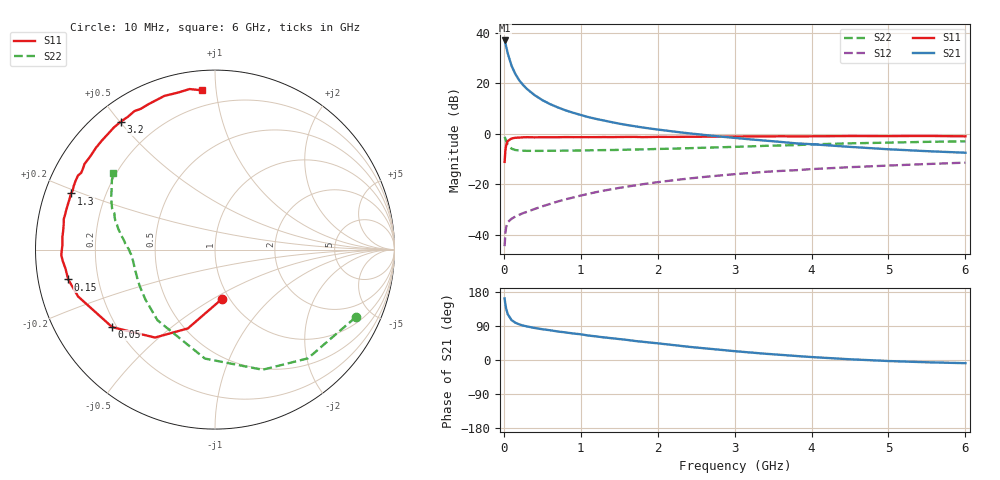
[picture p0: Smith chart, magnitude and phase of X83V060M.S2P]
! SIEMENS Small Signal Semiconductors
! BFP136W
! Si NPN RF Bipolar Junction Transistor in SOT343
! VCE = 3 V  IC = 60 mA
! Common Emitter S-Parameters:  September  1994
# GHz  S  MA  R  50
!  f  S11  S21  S12  S22
! GHz  MAG  ANG  MAG  ANG  MAG  ANG  MAG  ANG
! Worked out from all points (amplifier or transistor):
!   40 points, 10 MHz to 6 GHz, reference 50 ohm
!   highest |S21| = 36.9 dB at 10 MHz (marker M1)
!   |S21| within 3 dB of that: start of sweep to 34.86 MHz
!   unconditionally stable (mu >= 1): 594.7 MHz to 2.885 GHz
!   at 200 MHz: K = 0.59, MSG = 26.6 dB, |S12| = -32.0 dB
!   at 1.5 GHz: K = 1.10, MAG = 10.8 dB, |S12| = -21.4 dB
!   at 6 GHz: K = 0.96, MSG = 2.0 dB, |S12| = -11.4 dB
!   S11 on the Smith chart (normalised r, x): 10 MHz: 0.92, -0.55; 50 MHz: 0.18, -0.32; 150 MHz: 0.09, -0.10; 1.3 GHz: 0.08, +0.19; 3.2 GHz: 0.08, +0.50; 6 GHz: 0.11, +0.92
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0.01  0.278 -82.1  69.91 162.3  0.006 72.6  0.8694 -25.7
0.02  0.4645 -109.0  61.72 147.1  0.0108 60.3  0.7969 -49.5
0.03  0.5932 -124.3  53.35 135.8  0.0143 51.5  0.72 -68.4
0.05  0.7175 -143.0  39.19 121.1  0.0178 40.2  0.6097 -95.3
0.1  0.8063 -161.1  22.14 105.3  0.0209 33.4  0.5075 -129.2
0.15  0.8345 -168.5  15.15 98.3  0.0231 35.1  0.477 -144.5
0.2  0.8395 -172.7  11.41 94.0  0.025 36.7  0.4671 -152.8
0.25  0.851 -175.8  9.205 90.9  0.027 38.7  0.4632 -158.1
0.3  0.857 -178.0  7.703 88.6  0.0286 41.0  0.4599 -161.8
0.4  0.8504 178.1  5.804 84.5  0.0326 45.5  0.4592 -166.6
0.5  0.8532 175.3  4.629 81.2  0.0368 48.8  0.4596 -169.7
0.6  0.8524 173.2  3.864 78.5  0.041 51.5  0.4606 -171.7
0.7  0.8545 170.6  3.326 75.3  0.0458 53.9  0.4622 -173.1
0.9  0.8576 166.8  2.604 70.1  0.0549 56.1  0.4653 -175.7
1.1  0.8575 162.4  2.133 64.5  0.065 57.6  0.4703 -177.3
1.3  0.8614 158.7  1.829 59.7  0.0752 58.2  0.4756 -178.9
1.7  0.8676 151.6  1.411 50.3  0.095 57.2  0.4878 178.2
2.2  0.8674 143.3  1.109 39.5  0.1202 54.5  0.5076 174.6
3.2  0.8852 126.4  0.776 19.9  0.1677 46.0  0.5632 165.8
4.5  0.9016 108.2  0.551 1.9  0.2186 34.0  0.6467 153.5
5.5  0.9057 99.0  0.453 -6.0  0.2522 26.1  0.6923 146.1
6  0.89 94.6  0.422 -8.4  0.2688 21.7  0.7092 142.9
